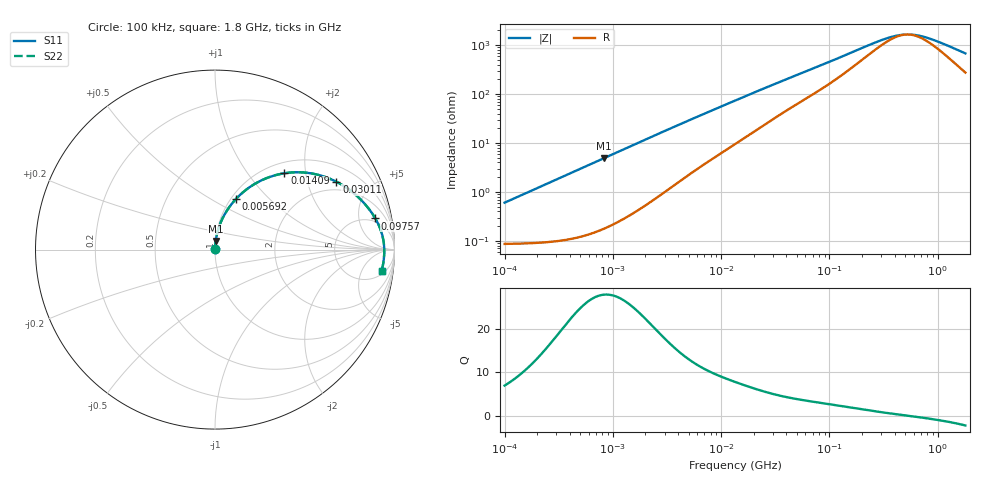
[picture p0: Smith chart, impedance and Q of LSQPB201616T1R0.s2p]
! LSQPB201616T1R0  S-PARAMETER MODEL  ( General Type )
! Model Generated by TAIYO YUDEN Corporation (http://www.ty-top.com)
! Version 3.0
! TAIYO YUDEN Control No. 130611NC14SB-FKC
! Copyright(c) 2008 TAIYO YUDEN CO.,LTD. All Rights Reserved.
! Product Description (link to TY-COMPAS)
! https://ds.yuden.co.jp/TYCOMPAS/or/detail?pn=LSQPB201616T1R0M&u=M
! Products Name : Inductors
! Characteristics :
!  Inductance : 1.0 uH , SRF(min) : 450 MHz , DC Resistance(max) : 0.1105 Ohm
!  Rated Current : Saturation :1350 mA , Temp Rise : 1100 mA (40 degC)
!  Case Size : 2.0 x 1.6 / 0.079 x 0.063 [mm/inch] , Thickness : 1.6 / 0.063 [mm/inch]
!  (Conditions: Temperature = 25 degC , DC Bias Current/Voltage = 0A / 0V)
! External Node Assignments :
!  1  o---GGG---o  2
! GND o---------o GND
! Frequency Range : 0.1MHz  -  1800MHz  [ 402 STEP ]
# MHz S RI R 50
! Freq[MHz].  S11 Real  S11 Imag  S21 Real  S21 Imag  S12 Real  S12 Imag  S22 Real  S22 Imag
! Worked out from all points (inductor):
!   401 points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, 100 kHz to 1.8 GHz, reference 50 ohm
!   read as one part in series: L = 950 nH near 105 kHz
!   highest Q = 27.8 at 822 kHz (marker M1), where L = 946 nH
!   self-resonance near 521.9 MHz
!   S11 on the Smith chart (normalised r, x): 100 kHz: 1.00, +0.01; 5.692 MHz: 1.05, +0.65; 14.09 MHz: 1.20, +1.53; 30.11 MHz: 1.61, +3.05; 97.57 MHz: 4.14, +8.36; 1.8 GHz: 7, -12
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0.1  0.0009 0.00596  0.9991 -0.00596  0.9991 -0.00596  0.0009 0.00596
0.516129  0.00217 0.0306  0.9978 -0.0306  0.9978 -0.0306  0.00217 0.0306
0.822022  0.00413 0.0486  0.9959 -0.0486  0.9959 -0.0486  0.00413 0.0486
1.55409  0.012 0.0904  0.988 -0.0904  0.988 -0.0904  0.012 0.0904
2.66389  0.0314 0.1501  0.9686 -0.1501  0.9686 -0.1501  0.0314 0.1501
4.039851  0.0653 0.2155  0.9347 -0.2155  0.9347 -0.2155  0.0653 0.2155
5.692459  0.1152 0.2804  0.8848 -0.2804  0.8848 -0.2804  0.1152 0.2804
8.632747  0.2139 0.3614  0.7861 -0.3614  0.7861 -0.3614  0.2139 0.3614
13.41641  0.3675 0.4219  0.6325 -0.4219  0.6325 -0.4219  0.3675 0.4219
14.09005  0.387 0.4254  0.613 -0.4254  0.613 -0.4254  0.387 0.4254
20.3463  0.5358 0.4247  0.4642 -0.4247  0.4642 -0.4247  0.5358 0.4247
30.10899  0.6763 0.3781  0.3237 -0.3781  0.3237 -0.3781  0.6763 0.3781
44.5561  0.7795 0.3087  0.2205 -0.3087  0.2205 -0.3087  0.7795 0.3087
69.24595  0.8556 0.2293  0.1444 -0.2293  0.1444 -0.2293  0.8556 0.2293
97.57284  0.8932 0.1737  0.1068 -0.1737  0.1068 -0.1737  0.8932 0.1737
171.3985  0.9267 0.0987  0.0733 -0.0987  0.0733 -0.0987  0.9267 0.0987
357.3983  0.9412 0.0292  0.0588 -0.0292  0.0588 -0.0292  0.9412 0.0292
491.4156  0.9429 0.00454  0.0571 -0.00454  0.0571 -0.00454  0.9429 0.00454
569.2172  0.9431 -0.00659  0.0569 0.00659  0.0569 0.00659  0.9431 -0.00659
675.6865  0.9429 -0.0198  0.0571 0.0198  0.0571 0.0198  0.9429 -0.0198
952.0939  0.9411 -0.0483  0.0589 0.0483  0.0589 0.0483  0.9411 -0.0483
1800  0.9287 -0.118  0.0713 0.118  0.0713 0.118  0.9287 -0.118
